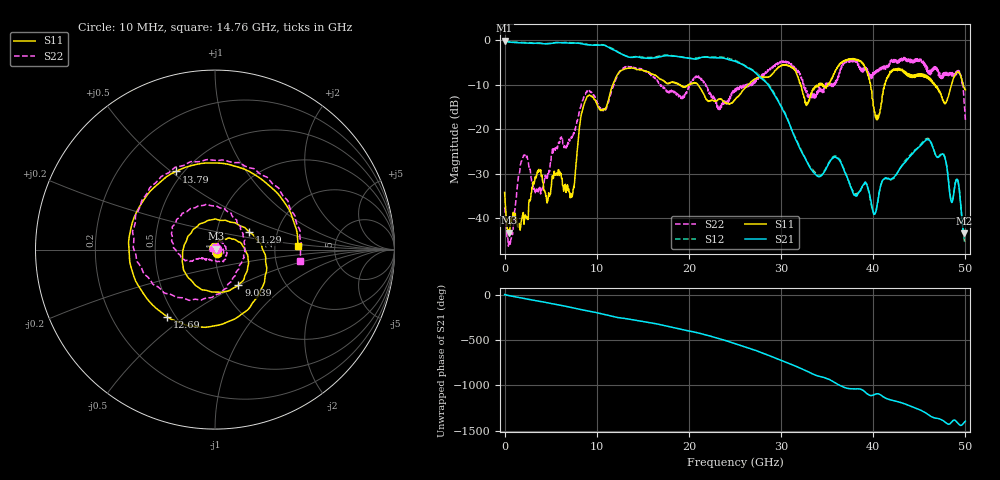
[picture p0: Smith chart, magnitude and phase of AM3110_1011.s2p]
# Hz S DB R 50.0
!freq dBS11 angS11 dBS21 angS21 dBS12 angS12 dBS22 angS22
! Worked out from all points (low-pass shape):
!   1601 points, 10 MHz to 50 GHz, reference 50 ohm
!   highest |S21| = -0.07 dB at 10 MHz (marker M1); lowest = -43.3 dB at 49.88 GHz (marker M2)
!   |S21| within 3 dB of the highest: start of sweep to 12.65 GHz
!   lowest |S11| = -43.2 dB at 509.9 MHz (marker M3), VSWR 1.01, Z = 50.4 + j0.553 ohm
!   |S11| at or under -10 dB: start of sweep to 11.76 GHz; 20.99 GHz to 26.45 GHz (5.454 GHz wide, 23 % of centre); 32.12 GHz to 34.07 GHz (1.951 GHz wide, 5.89 % of centre)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
!   |S22| runs from -46.2 to -3.8 dB; largest |S21 - S12| = 0.026
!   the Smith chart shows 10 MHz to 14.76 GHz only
!   S11 on the Smith chart (normalised r, x): 10 MHz: 1.02, -0.04; 9.039 GHz: 1.19, -0.50; 11.29 GHz: 1.44, +0.30; 12.69 GHz: 0.45, -0.43; 13.79 GHz: 0.46, +0.52; 14.76 GHz: 2.72, +0.14
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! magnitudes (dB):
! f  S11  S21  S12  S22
! 10 MHz  -34.2  -0.1  -0.1  -37.5
! 509.9 MHz  -43.2  -0.4  -0.3  -45.7
! 1.978 GHz  -39.2  -0.6  -0.5  -26.4
! 3.79 GHz  -29.4  -0.6  -0.7  -33.8
! 7.29 GHz  -35.3  -0.7  -0.6  -22.0
! 8.352 GHz  -16.4  -0.8  -0.6  -14.2
! 9.039 GHz  -12.5  -1.0  -1.0  -11.5
! 11.29 GHz  -13.4  -1.6  -1.5  -13.9
! 12.69 GHz  -6.8  -3.1  -3.1  -6.5
! 13.79 GHz  -6.3  -3.9  -3.8  -6.0
! 14.76 GHz  -6.7  -3.9  -3.7  -6.4
! 16.69 GHz  -8.4  -3.8  -3.6  -9.5
! 25 GHz  -13.4  -4.7  -4.5  -11.3
! 30.38 GHz  -5.5  -16.4  -16.2  -4.7
! 33.35 GHz  -11.7  -29.2  -28.8  -12.9
! 38.38 GHz  -4.4  -34.4  -34.3  -5.2
! 40.47 GHz  -17.8  -36.4  -36.5  -7.0
! 41.69 GHz  -7.8  -31.0  -31.2  -5.9
! 46.03 GHz  -8.6  -22.4  -22.1  -6.5
! 49.16 GHz  -7.1  -31.4  -31.4  -7.5
! 49.88 GHz  -10.7  -43.3  -44.9  -14.4
! 50 GHz  -11.1  -43.0  -45.7  -17.9
